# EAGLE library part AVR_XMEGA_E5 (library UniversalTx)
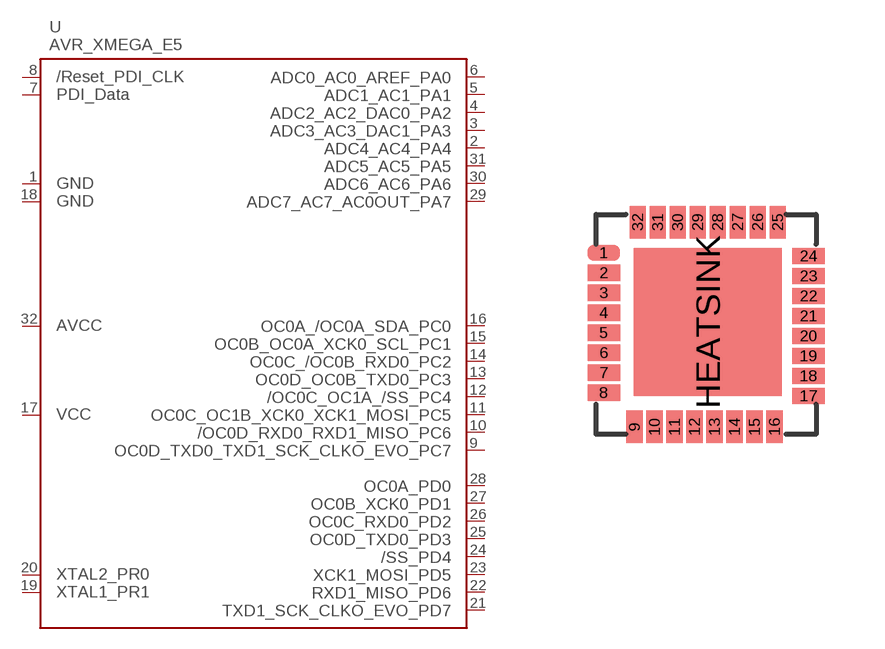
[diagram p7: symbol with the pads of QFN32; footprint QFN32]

Designator prefix -

## AVR_XMEGA_E5  [QFN32]
1  GND1
2  PA4
3  PA3
4  PA2
5  PA1
6  PA0
7  PDI_DATA
8  RESET
9  PC7
10  PC6
11  PC5
12  PC4
13  PC3
14  PC2
15  PC1
16  PC0
17  VCC1
18  GND2
19  PR1
20  PR0
21  PD7
22  PD6
23  PD5
24  PD4
25  PD3
26  PD2
27  PD1
28  PD0
29  PA7
30  PA6
31  PA5
32  AVCC

## Footprint QFN32 (pad centres in mm)
smd 0.813 x 0.406: 1 -2.56,1.79; 2 -2.56,1.29; 3 -2.56,0.79; 4 -2.56,0.29; 5 -2.56,-0.21; 6 -2.56,-0.71; 7 -2.56,-1.21; 8 -2.56,-1.71; 17 2.56,-1.79; 18 2.56,-1.29; 19 2.56,-0.79; 20 2.56,-0.29; 21 2.56,0.21; 22 2.56,0.71; 23 2.56,1.21; 24 2.56,1.71
smd 0.406 x 0.813: 9 -1.79,-2.56; 10 -1.29,-2.56; 11 -0.79,-2.56; 12 -0.29,-2.56; 13 0.21,-2.56; 14 0.71,-2.56; 15 1.21,-2.56; 16 1.71,-2.56; 25 1.79,2.56; 26 1.29,2.56; 27 0.79,2.56; 28 0.29,2.56; 29 -0.21,2.56; 30 -0.71,2.56; 31 -1.21,2.56; 32 -1.71,2.56
smd 3.7 x 3.7: HEATSINK 0.04,0.06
